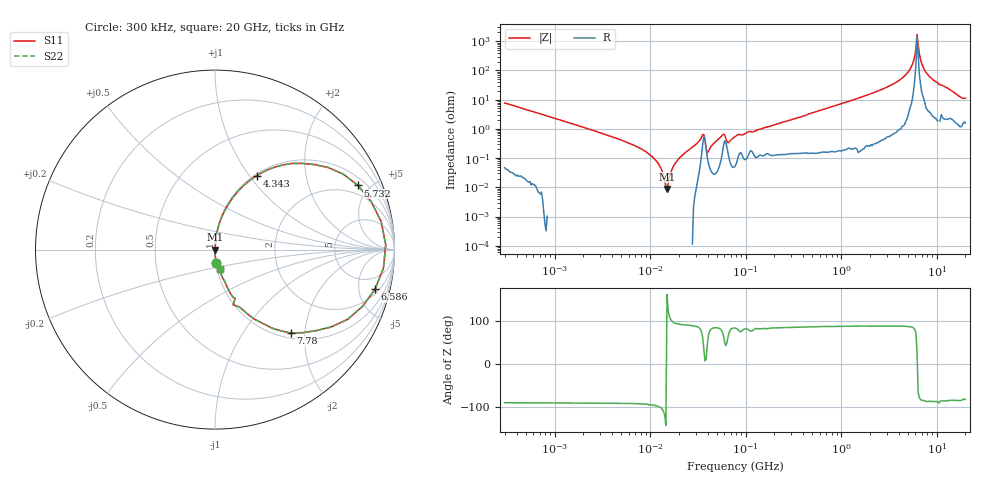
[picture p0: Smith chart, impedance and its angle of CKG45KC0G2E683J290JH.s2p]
! S-Parameter Data Generated by TDK Corporation
! Copyright(C) 2022 TDK Corporation.
! All Rights Reserved.
! TDK P/N: CKG45KC0G2E683J290JH (Multilayer Ceramic Chip Capacitor)
! Property: C=68nF
! Size(LxWxT): 5x3.5x2.9mm
! Model Type: s2p (Touchstone File Format Version 1.0)
! Frequency: DC=Yes Start=0.3MHz Stop=20000MHz 402points Log-sweep
! Model Generated on Apr. 15, 2022
! Port Assignments:
!  1 ---| |--- 2
! Applicable Conditions:
!  Temperature = 25 degC
!  DC Bias Voltage = 0 V
!  Small Signal Operation
! Terms and conditions regarding TDK Simulation Models
! (1)This simulation model is being provided solely for informational purposes. Please refer to the specifications of the products in terms of detailed characteristics of such products.
! (2)In no event shall TDK Corporation of any of its subsidiaries be liable for any loss or damage arising, directly or indirectly,
!  From any information contained in this simulation model, including, but not limited to loss or damages arising from any inaccuracies, omissions or errors in connection with such information.
! (3)Any and all copyrights on this simulation model are owned by TDK Corporation.
!  Duplication or redistribution of this simulation model without prior written permission from TDK Corporation is prohibited.
! (4)This simulation model is subject to any modification or change without any prior notice.
! (5)Neither TDK Corporation nor any of its subsidiaries shall make any warranty, express or implied,
!  Including but not limited to the correctness, implied warranties of merchantability and fitness for a particular purpose with respect to this simulation models.
! (6)The use of this simulation model shall be deemed to have consented to the terms and conditions hereof.
# Hz S MA R 50
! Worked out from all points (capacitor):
!   401 points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, 300 kHz to 20 GHz, reference 50 ohm
!   read as one part in series: C = 68.4 nF near 317.1 kHz
!   lowest |Z| = 8.8 mohm at 15.05 MHz (marker M1)
!   series resonance near 14.93 MHz, so ESL is about 1.7 nH
!   S11 on the Smith chart (normalised r, x): 300 kHz: 1.00, -0.15; 4.343 GHz: 1.02, +1.09; 5.732 GHz: 1.41, +4.23; 6.586 GHz: 2.57, -7.27; 7.78 GHz: 1.10, -1.69; 20 GHz: 1.03, -0.22
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300000  0.07716 -85.2  0.9965 4.4  0.9965 4.4  0.07716 -85.2
1928084  0.01181 -89.8  1 0.7  1 0.7  0.01181 -89.8
7311307  0.002439 -91.8  1 0.1  1 0.1  0.002439 -91.8
1.239169e7  0.0005967 -98.9  1 0.0  1 0.0  0.0005967 -98.9
1.505044e7  8.802e-05 162.6  1 -0.0  1 -0.0  8.802e-05 162.6
1.932356e7  0.0008386 94.4  1 -0.0  1 -0.0  0.0008386 94.4
3.462121e7  0.005259 75.4  0.9987 -0.3  0.9987 -0.3  0.005259 75.4
4.089789e7  0.001752 68.4  0.9994 -0.1  0.9994 -0.1  0.001752 68.4
5.707135e7  0.006017 75.5  0.9985 -0.3  0.9985 -0.3  0.006017 75.5
6.741814e7  0.003608 74.9  0.9991 -0.2  0.9991 -0.2  0.003608 74.9
7.964076e7  0.005812 83.5  0.9994 -0.3  0.9994 -0.3  0.005812 83.5
4.978292e8  0.03526 85.6  0.9979 -2.0  0.9979 -2.0  0.03526 85.6
3.199522e9  0.2809 72.6  0.9546 -16.3  0.9546 -16.3  0.2809 72.6
4.342527e9  0.4734 60.5  0.8703 -28.3  0.8703 -28.3  0.4734 60.5
5.274253e9  0.7292 40.5  0.65 -46.7  0.65 -46.7  0.7292 40.5
5.73245e9  0.8728 24.2  0.4111 -60.3  0.4111 -60.3  0.8728 24.2
6.059821e9  0.9388 9.6  0.1735 -64.6  0.1735 -64.6  0.9388 9.6
6.586264e9  0.9183 -14.0  0.2468 63.8  0.2468 63.8  0.9183 -14.0
6.962395e9  0.8351 -27.7  0.4683 56.1  0.4683 56.1  0.8351 -27.7
7.780325e9  0.6272 -47.8  0.7424 38.8  0.7424 38.8  0.6272 -47.8
1.027059e10  0.3492 -66.8  0.92 20.4  0.92 20.4  0.3492 -66.8
2e10  0.1099 -75.7  0.9787 6.2  0.9787 6.2  0.1099 -75.7
